FUNCTION_BLOCK ReadFileOnDisk	//Opens, reads, then closes a file on disk
VAR_INPUT
	Execute : BOOL;	//Execution of the function block begins on a rising edge of this input
	file_path : STRING(255);	//Location of the file on the disk
	buffer_size : UDINT := 500000;	//Number of bytes available in the buffer 
END_VAR
VAR_OUTPUT
	Done : BOOL;	//Function block is finished, any returned values can be used
	file_size : DINT;	//Amount of data read from the file
END_VAR
VAR_IN_OUT
	data : ARRAY[*] OF SINT;	//data read from the file as a raw binary
END_VAR
VAR
	file_open : FB_FileOpen;
	file_read : FB_FileRead;
	file_close : FB_FileClose;
END_VAR

file_open(sNetId := '',sPathName := file_path,nMode := FOPEN_MODEREAD OR FOPEN_MODEBINARY,ePath := PATH_GENERIC,bExecute := Execute,tTimeout := T#10S);

file_read(sNetId := '',hFile := file_open.hFile,pReadBuff := data,cbReadLen := buffer_size,bExecute := file_open.bExecute AND NOT(file_open.bBusy) AND NOT(file_open.bError),tTimeout := T#10S);
file_size := file_read.cbRead;

file_close(sNetId := '',hFile := file_open.hFile,bExecute := file_read.bExecute AND NOT(file_read.bBusy) AND NOT(file_read.bError),tTimeout := T#10S);

Done := file_close.bExecute AND NOT(file_close.bBusy) AND NOT(file_close.bError);

END_FUNCTION_BLOCK
